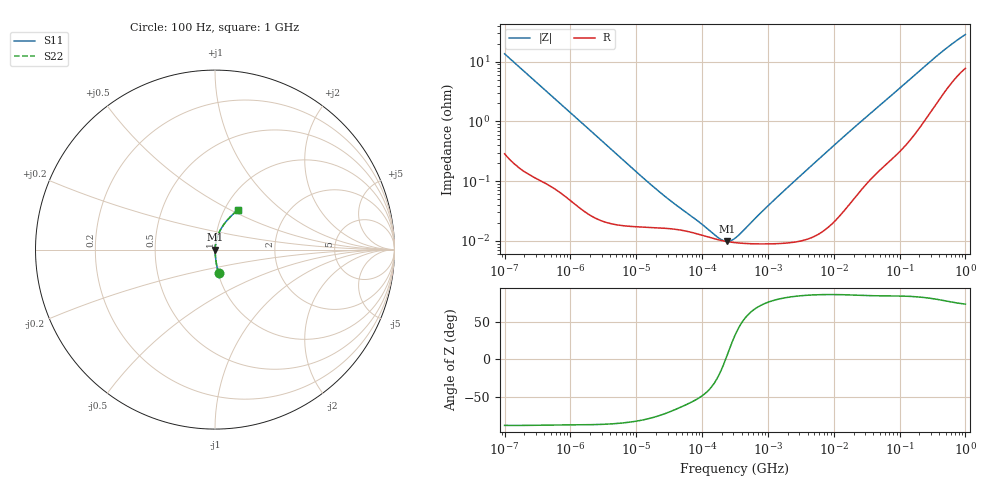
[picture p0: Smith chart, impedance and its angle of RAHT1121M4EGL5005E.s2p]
! RAHT1121M4EGL5005E  S-PARAMETER MODEL  (AEC-Q200 qualified)
! Model Generated by ELNA Corporation (http://www.ty-top.com)
! Version 1.0
! ELNA Control No. 201214
! Copyright (c) 2020 ELNA CO.,LTD. All Rights Reserved.
! Products Name : CONDUCTIVE POLYMER HYBRID ALUMINUM ELECTROLYTIC CAPACITORS
! Characteristics :
!  Capacitance  :  120uF  ,  Rated voltage  :  63V
!  Operating Temp. Range  :  -55 to +105 degC  ,  Endurance  :  10000hr at 105 degC
!  Dimension D  :  12.5mm  ,  Dimension L  :  13.5mm
! Frequency Range : 100Hz - 1GHz
! External Node Assignments :
!  1  o---| |---o  2
# MHz S RI R 50
!Freq[MHz].  S11 Real  S11 Imag  S21 Real  S21 Imag  S12 Real  S12 Imag  S22 Real  S22 Imag
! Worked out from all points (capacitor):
!   401 points, 100 Hz to 1 GHz, reference 50 ohm
!   read as one part in series: C = 117 uF near 108 Hz
!   lowest |Z| = 9.78 mohm at 238.5 kHz (marker M1)
!   series resonance near 227.7 kHz, so ESL is about 4.2 nH
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0.0001  0.0209 -0.1327  0.9791 0.1327  0.9791 0.1327  0.0209 -0.1327
0.000113  0.0167 -0.1182  0.9833 0.1182  0.9833 0.1182  0.0167 -0.1182
0.000309  0.00304 -0.0441  0.997 0.0441  0.997 0.0441  0.00304 -0.0441
0.001488  0.000424 -0.00946  0.9996 0.00946  0.9996 0.00946  0.000424 -0.00946
0.009495  0.000175 -0.0015  0.9998 0.0015  0.9998 0.0015  0.000175 -0.0015
0.022131  0.000166 -0.000651  0.9998 0.000651  0.9998 0.000651  0.000166 -0.000651
0.037368  0.000157 -0.000394  0.9998 0.000394  0.9998 0.000394  0.000157 -0.000394
0.090678  0.000128 -0.000161  0.9999 0.000161  0.9999 0.000161  0.000128 -0.000161
0.172783  0.000105 -4.72e-05  0.9999 4.72e-05  0.9999 4.72e-05  0.000105 -4.72e-05
0.203002  0.000101 -1.97e-05  0.9999 1.97e-05  0.9999 1.97e-05  0.000101 -1.97e-05
0.238506  9.74e-05 8.06e-06  0.9999 -8.06e-06  0.9999 -8.06e-06  9.74e-05 8.06e-06
0.280221  9.49e-05 3.67e-05  0.9999 -3.67e-05  0.9999 -3.67e-05  9.49e-05 3.67e-05
0.316228  9.34e-05 5.9e-05  0.9999 -5.9e-05  0.9999 -5.9e-05  9.34e-05 5.9e-05
0.386812  9.15e-05 9.87e-05  0.9999 -9.87e-05  0.9999 -9.87e-05  9.15e-05 9.87e-05
1.102808  8.93e-05 0.000418  0.9999 -0.000418  0.9999 -0.000418  8.93e-05 0.000418
4.704354  0.000118 0.00186  0.9999 -0.00186  0.9999 -0.00186  0.000118 0.00186
18.51399  0.000499 0.0072  0.9995 -0.0072  0.9995 -0.0072  0.000499 0.0072
69.9842  0.00277 0.0253  0.9972 -0.0253  0.9972 -0.0253  0.00277 0.0253
169.8244  0.00954 0.0588  0.9905 -0.0588  0.9905 -0.0588  0.00954 0.0588
380.1894  0.0359 0.12  0.9641 -0.12  0.9641 -0.12  0.0359 0.12
641.9482  0.0775 0.1742  0.9225 -0.1742  0.9225 -0.1742  0.0775 0.1742
1000  0.1291 0.2228  0.8709 -0.2228  0.8709 -0.2228  0.1291 0.2228
